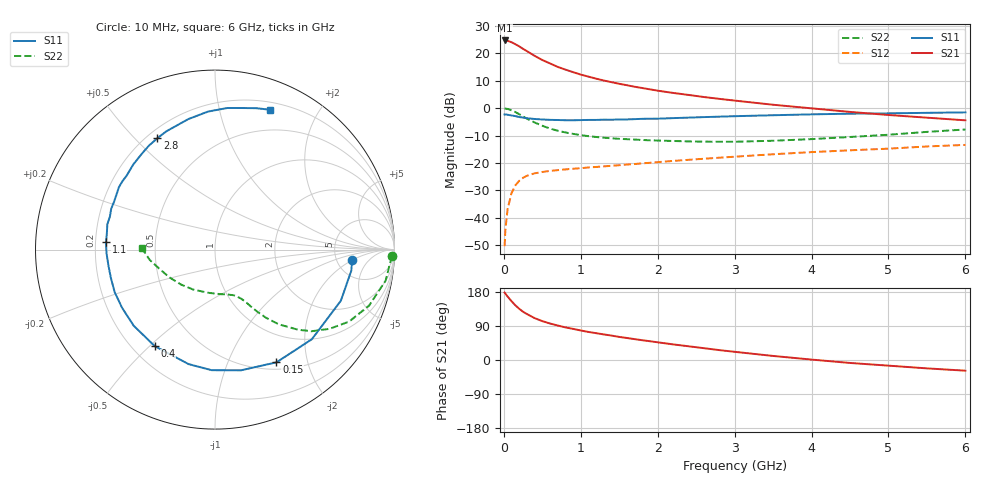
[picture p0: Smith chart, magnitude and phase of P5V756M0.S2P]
! SIEMENS Small Signal Semiconductors
! BFP183
! Si NPN RF Bipolar Junction Transistor in SOT143
! VCE = 0.75 V  IC = 6 mA
! Common Emitter S-Parameters:  March  1996
# GHz  S  MA  R  50
!  f  S11  S21  S12  S22
! GHz  MAG  ANG  MAG  ANG  MAG  ANG  MAG  ANG
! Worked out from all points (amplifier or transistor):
!   36 points, 10 MHz to 6 GHz, reference 50 ohm
!   highest |S21| = 24.7 dB at 10 MHz (marker M1)
!   |S21| within 3 dB of that: start of sweep to 246.1 MHz
!   unconditionally stable (mu >= 1): 1.315 GHz to end of sweep
!   at 250 MHz: K = 0.25, MSG = 23.6 dB, |S12| = -25.5 dB
!   at 1.4 GHz: K = 1.05, MAG = 14.0 dB, |S12| = -21.1 dB
!   at 6 GHz: K = 1.07, MAG = 2.9 dB, |S12| = -13.4 dB
!   S11 on the Smith chart (normalised r, x): 10 MHz: 6.98, -1.99; 150 MHz: 0.59, -1.52; 400 MHz: 0.29, -0.52; 1.1 GHz: 0.24, +0.03; 2.8 GHz: 0.24, +0.58; 6 GHz: 0.27, +1.43
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0.01  0.7664 -4.4  17.27 177.7  0.003 88.0  0.9863 -2.1
0.02  0.7684 -8.8  17.24 175.3  0.006 88.4  0.9791 -4.2
0.05  0.7569 -22.1  17 167.1  0.0146 80.2  0.9664 -10.3
0.1  0.7352 -42.8  16.02 155.1  0.0281 69.0  0.9133 -20.0
0.15  0.7155 -61.4  14.76 144.3  0.0388 60.8  0.8482 -28.2
0.2  0.6879 -77.9  13.48 135.1  0.047 54.0  0.7758 -34.7
0.25  0.6721 -91.6  12.13 127.3  0.0533 48.2  0.7047 -40.2
0.3  0.6547 -103.0  11 121.3  0.0581 44.5  0.6425 -44.0
0.4  0.6339 -122.0  9.045 110.5  0.0644 38.5  0.5475 -49.5
0.5  0.6206 -136.9  7.585 102.6  0.0681 34.7  0.4762 -53.1
0.6  0.6108 -148.1  6.568 96.3  0.0713 32.2  0.424 -55.5
0.7  0.6071 -157.1  5.682 91.0  0.0736 31.1  0.3866 -57.2
0.8  0.6011 -165.0  5.067 86.1  0.0759 30.0  0.3597 -58.5
1.1  0.6091 176.0  3.767 74.0  0.0824 29.3  0.3077 -62.2
1.5  0.6215 158.5  2.79 60.9  0.0906 29.7  0.2746 -67.8
1.8  0.6384 147.0  2.331 52.2  0.0979 30.1  0.262 -73.1
2.2  0.6573 133.9  1.899 41.2  0.1084 29.8  0.2512 -81.8
2.8  0.6987 117.3  1.48 26.1  0.1243 28.6  0.2435 -97.7
3.5  0.7421 101.6  1.154 10.7  0.1437 25.7  0.2536 -118.6
4.5  0.792 85.0  0.854 -7.8  0.1696 19.8  0.2972 -148.6
5.5  0.8212 73.6  0.67 -22.1  0.1994 14.0  0.3683 -171.1
6  0.8373 68.5  0.599 -28.2  0.2129 9.9  0.4075 179.0
